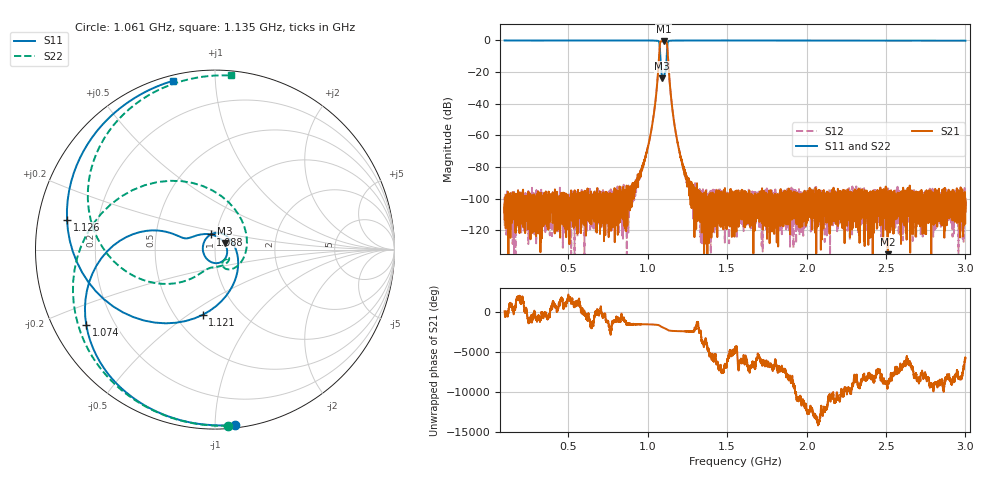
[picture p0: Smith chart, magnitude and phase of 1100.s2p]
# Hz S DB R 50
! Planar, S50180, 20087770, 20.1.2/1
! Date: 23.06.2021 14:41:37
! Data: Format (Calibration Info)
! Freq	S11:dB/Ang(F2)	S21:dB/Ang(F2)	S12:dB/Ang(F2)	S22:dB/Ang(F2)
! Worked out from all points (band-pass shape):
!   8991 points, 100 MHz to 3 GHz, reference 50 ohm
!   highest |S21| = -0.45 dB at 1.101 GHz (marker M1); lowest = -142.1 dB at 2.513 GHz (marker M2)
!   |S21| within 3 dB of the highest: 1.076 GHz to 1.123 GHz (46.83 MHz wide, 4.26 % of centre)
!   lowest |S11| = -23.9 dB at 1.091 GHz (marker M3), VSWR 1.14, Z = 55.4 + j4 ohm
!   |S11| at or under -10 dB: 1.08 GHz to 1.12 GHz (40.39 MHz wide, 3.67 % of centre)
!   |S22| runs from -22.2 to 0.0 dB; largest |S21 - S12| = 0.003
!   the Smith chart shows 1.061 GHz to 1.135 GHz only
!   S11 on the Smith chart (normalised r, x): 1.061 GHz: 0.02, -1.12; 1.074 GHz: 0.10, -0.27; 1.088 GHz: 0.94, +0.16; 1.121 GHz: 0.68, -0.57; 1.126 GHz: 0.09, +0.10; 1.135 GHz: 0.03, +0.78
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1e8  0.02 154.1  -108.77 77.6  -100.66 152.0  0.01 150.3
3.148387e8  -0.03 103.6  -98.52 171.9  -102.84 39.5  -0.00 95.0
5.835484e8  -0.01 54.0  -104.22 50.9  -99.18 -81.9  0.01 44.8
9.63871e8  0.01 -10.9  -81.22 -100.6  -81.57 -98.3  0.02 -16.1
1.020968e9  -0.02 -34.1  -58.09 -127.3  -58.05 -127.4  0.00 -37.4
1.060645e9  -0.15 -83.4  -26.81 -177.4  -26.82 -177.6  -0.14 -85.7
1.066774e9  -0.29 -104.0  -18.64 160.2  -18.65 159.9  -0.33 -108.7
1.073871e9  -1.60 -149.5  -7.12 106.9  -7.12 106.7  -1.83 -167.3
1.088065e9  -21.14 106.2  -0.52 -72.2  -0.53 -72.3  -19.70 -64.6
1.090968e9  -23.87 34.1  -0.48 -99.8  -0.49 -100.0  -22.08 -53.8
1.100968e9  -23.50 -162.5  -0.45 171.2  -0.46 171.1  -21.68 -31.7
1.120645e9  -8.64 -100.6  -1.49 -30.8  -1.49 -30.9  -8.44 -150.3
1.126452e9  -1.51 168.7  -7.88 -111.0  -7.88 -111.1  -1.41 141.0
1.135484e9  -0.27 104.1  -21.85 -172.4  -21.85 -172.5  -0.23 84.9
1.146129e9  -0.12 72.4  -34.47 156.8  -34.47 156.6  -0.11 56.6
1.174194e9  -0.04 37.7  -56.53 123.1  -56.46 122.8  -0.05 25.5
1.22871e9  -0.03 12.7  -81.27 99.3  -81.29 92.4  0.02 3.5
1.55e9  -0.01 -32.6  -100.33 145.4  -100.51 44.2  0.03 -37.6
2.033548e9  -0.04 -72.6  -109.69 -7.9  -113.52 -97.8  -0.01 -74.2
2.512581e9  -0.08 -108.0  -142.07 73.6  -100.60 45.3  -0.06 -106.7
2.516774e9  -0.07 -108.3  -102.83 -105.3  -101.05 -163.1  -0.05 -107.0
3e9  -0.11 -145.0  -99.99 -6.0  -103.67 5.8  -0.10 -140.9
